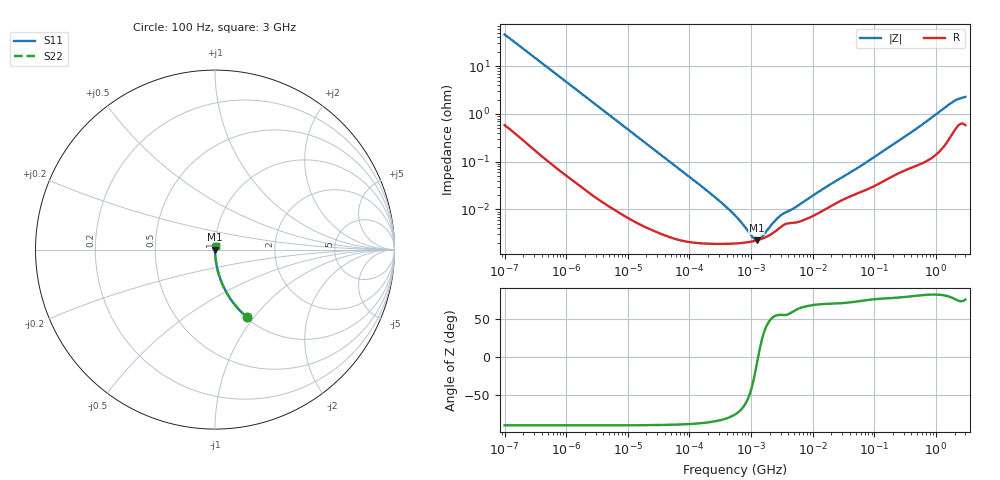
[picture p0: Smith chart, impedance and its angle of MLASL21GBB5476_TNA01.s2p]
! MLASL21GBB5476_TNA01  S-PARAMETER MODEL  ( Standard Model )
! Model Generated by TAIYO YUDEN Corporation (http://www.ty-top.com)
! Version 1.0
! TAIYO YUDEN Control No. 220601
! Copyright(c) 2016 TAIYO YUDEN CO.,LTD. All Rights Reserved.
! Product Description (link to TY-COMPAS)
! https://ds.yuden.co.jp/TYCOMPAS/or/detail?pn=MLASL21GBB5476MTNA01&u=M
! Products Name : Multilayer Ceramic Capacitors
! Characteristics :
!  Capacitance : 47 [uF] , Rated Voltage : 10 [V] , TCC : X5R
!  Case Size : 2.0 x 1.25 / 0.079 x 0.049 [mm/inch] , Thickness : 1.25 / 0.049 [mm/inch]
!  (Conditions: Temperature = 25 [degC] , DC Bias Voltage = 0 [V])
! External Node Assignments :
!  1  o---| |---o  2
! GND o---------o GND
! Frequency Range : 100Hz  -  3GHz  [ 401 STEP ]
# MHZ S RI R 50
! Freq[MHz].  S11 Real  S11 Imag  S21 Real  S21 Imag  S12 Real  S12 Imag  S22 Real  S22 Imag
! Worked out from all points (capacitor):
!   401 points, 100 Hz to 3 GHz, reference 50 ohm
!   read as one part in series: C = 34.3 uF near 109 Hz
!   lowest |Z| = 2.28 mohm at 1.241 MHz (marker M1)
!   series resonance near 1.299 MHz, so ESL is about 440 pH
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0.0001  0.1794 -0.3774  0.8206 0.3774  0.8206 0.3774  0.1794 -0.3774
0.000114  0.1453 -0.3462  0.8547 0.3462  0.8547 0.3462  0.1453 -0.3462
0.000175  0.0686 -0.2467  0.9314 0.2467  0.9314 0.2467  0.0686 -0.2467
0.000348  0.0191 -0.1314  0.9809 0.1314  0.9809 0.1314  0.0191 -0.1314
0.000724  0.00488 -0.0645  0.9951 0.0645  0.9951 0.0645  0.00488 -0.0645
0.001788  0.000987 -0.0264  0.999 0.0264  0.999 0.0264  0.000987 -0.0264
0.031977  3.43e-05 -0.00151  1 0.00151  1 0.00151  3.43e-05 -0.00151
0.171338  1.94e-05 -0.000278  1 0.000278  1 0.000278  1.94e-05 -0.000278
0.405239  1.9e-05 -0.000108  1 0.000108  1 0.000108  1.9e-05 -0.000108
0.461094  1.91e-05 -9.17e-05  1 9.17e-05  1 9.17e-05  1.91e-05 -9.17e-05
0.547723  1.93e-05 -7.26e-05  1 7.26e-05  1 7.26e-05  1.93e-05 -7.26e-05
1.240863  2.25e-05 -3.33e-06  1 3.33e-06  1 3.33e-06  2.25e-05 -3.33e-06
4.513443  5.19e-05 8.41e-05  0.9999 -8.41e-05  0.9999 -8.41e-05  5.19e-05 8.41e-05
5.135543  5.29e-05 9.54e-05  0.9999 -9.54e-05  0.9999 -9.54e-05  5.29e-05 9.54e-05
9.794414  7.16e-05 0.000177  0.9999 -0.000177  0.9999 -0.000177  7.16e-05 0.000177
18.67973  0.000113 0.000306  0.9999 -0.000306  0.9999 -0.000306  0.000113 0.000306
59.714  0.000231 0.000777  0.9998 -0.000777  0.9998 -0.000777  0.000231 0.000777
175.1444  0.000458 0.00198  0.9995 -0.00198  0.9995 -0.00198  0.000458 0.00198
513.708  0.000877 0.00513  0.9991 -0.00513  0.9991 -0.00513  0.000877 0.00513
1789.813  0.00386 0.0168  0.9961 -0.0168  0.9961 -0.0168  0.00386 0.0168
2219.584  0.00579 0.0193  0.9942 -0.0193  0.9942 -0.0193  0.00579 0.0193
3000  0.00625 0.0218  0.9938 -0.0218  0.9938 -0.0218  0.00625 0.0218
